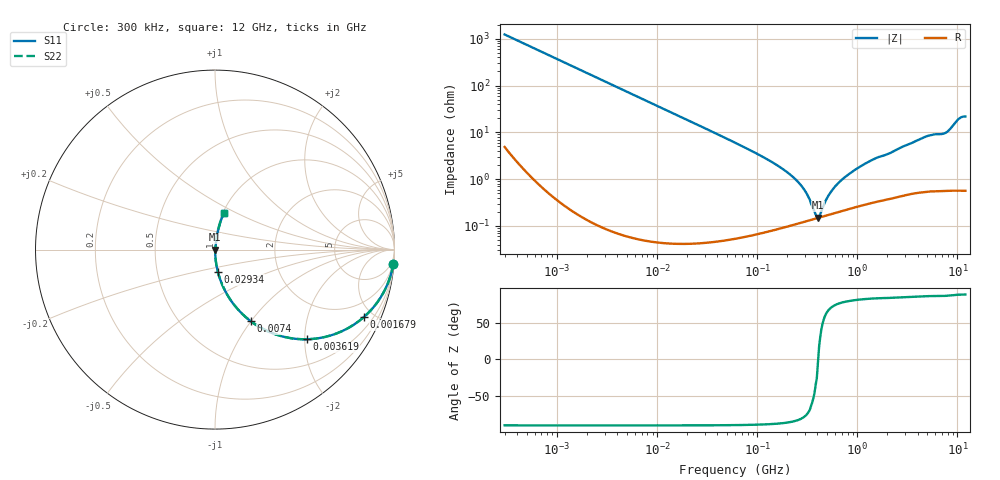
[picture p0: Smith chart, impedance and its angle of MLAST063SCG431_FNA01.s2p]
! MLAST063SCG431_FNA01  S-PARAMETER MODEL  ( General Type )
! Model Generated by TAIYO YUDEN Corporation (http://www.ty-top.com)
! Version 1.0
! TAIYO YUDEN Control No. 160830
! Copyright(c) 2016 TAIYO YUDEN CO.,LTD. All Rights Reserved.
! Product Description (link to TY-COMPAS)
! https://ds.yuden.co.jp/TYCOMPAS/or/detail?pn=MLAST063SCG431JFNA01&u=M
! Products Name : Multilayer Ceramic Capacitors
! Characteristics :
!  Capacitance : 430 pF , Rated Voltage : 25V , TCC : CG / C0G
!  Case Size : 0.6 x 0.3 / 0.024 x 0.012 [mm/inch] , Thickness : 0.3 / 0.012 [mm/inch]
!  (Conditions: Temperature = 25 degC , DC Bias Current/Voltage = 0A / 0V)
! External Node Assignments :
!  1  o---| |---o  2
! GND o---------o GND
! Frequency Range : 0.3MHz  -  12000MHz  [ 401 STEP ]
# MHz S RI R 50
! Freq[MHz].  S11 Real  S11 Imag  S21 Real  S21 Imag  S12 Real  S12 Imag  S22 Real  S22 Imag
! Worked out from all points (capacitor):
!   401 points, 300 kHz to 12 GHz, reference 50 ohm
!   read as one part in series: C = 431 pF near 316.3 kHz
!   lowest |Z| = 149 mohm at 404.1 MHz (marker M1)
!   series resonance near 406.4 MHz, so ESL is about 360 pH
!   S11 on the Smith chart (normalised r, x): 300 kHz: 1, -25; 1.679 MHz: 1.00, -4.40; 3.619 MHz: 1.00, -2.04; 7.4 MHz: 1.00, -1.00; 29.34 MHz: 1.00, -0.25; 12 GHz: 1.01, +0.44
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0.3  0.9931 -0.0806  0.00686 0.0806  0.00686 0.0806  0.9931 -0.0806
0.842989  0.9503 -0.2167  0.0497 0.2167  0.0497 0.2167  0.9503 -0.2167
1.678634  0.8288 -0.3763  0.1712 0.3763  0.1712 0.3763  0.8288 -0.3763
1.769972  0.8133 -0.3893  0.1867 0.3893  0.1867 0.3893  0.8133 -0.3893
3.61914  0.5105 -0.4995  0.4895 0.4995  0.4895 0.4995  0.5105 -0.4995
7.400216  0.1998 -0.3994  0.8002 0.3994  0.8002 0.3994  0.1998 -0.3994
10.44266  0.1115 -0.3141  0.8885 0.3141  0.8885 0.3141  0.1115 -0.3141
29.34352  0.0159 -0.1233  0.9841 0.1233  0.9841 0.1233  0.0159 -0.1233
60  0.00414 -0.06  0.9959 0.06  0.9959 0.06  0.00414 -0.06
213.9924  0.00116 -0.0124  0.9988 0.0124  0.9988 0.0124  0.00116 -0.0124
294.0765  0.00126 -0.00589  0.9987 0.00589  0.9987 0.00589  0.00126 -0.00589
353.9943  0.00137 -0.00227  0.9986 0.00227  0.9986 0.00227  0.00137 -0.00227
404.1309  0.00149 -0.000129  0.9985 0.000129  0.9985 0.000129  0.00149 -0.000129
426.1204  0.00154 0.000908  0.9985 -0.000908  0.9985 -0.000908  0.00154 0.000908
526.7124  0.00177 0.00447  0.9982 -0.00447  0.9982 -0.00447  0.00177 0.00447
704.9044  0.00219 0.00958  0.9978 -0.00958  0.9978 -0.00958  0.00219 0.00958
1197.383  0.0033 0.0212  0.9967 -0.0212  0.9967 -0.0212  0.0033 0.0212
2088.533  0.00497 0.035  0.995 -0.035  0.995 -0.035  0.00497 0.035
4875.354  0.0118 0.0803  0.9882 -0.0803  0.9882 -0.0803  0.0118 0.0803
7448.838  0.0144 0.0935  0.9856 -0.0935  0.9856 -0.0935  0.0144 0.0935
10236.47  0.0407 0.1833  0.9593 -0.1833  0.9593 -0.1833  0.0407 0.1833
12000  0.0503 0.206  0.9497 -0.206  0.9497 -0.206  0.0503 0.206
